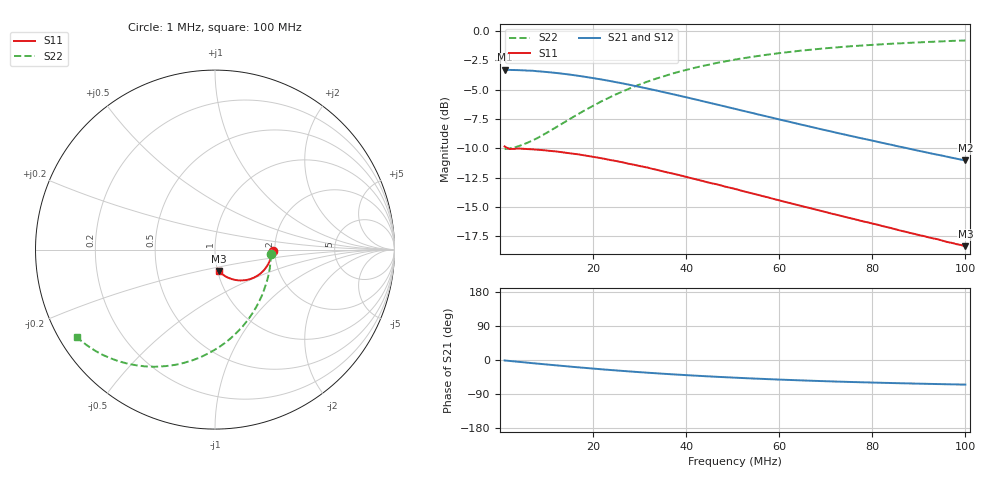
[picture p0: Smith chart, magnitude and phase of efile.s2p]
# Hz S RI R 50.0
! written by SimSmith version 18.3b
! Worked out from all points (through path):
!   101 points, 1 MHz to 100 MHz, reference 50 ohm
!   highest |S21| = -3.30 dB at 1 MHz (marker M1); lowest = -11.0 dB at 100 MHz (marker M2)
!   group delay of S21, straight-line fit = 1.73 ns
!   lowest |S11| = -18.3 dB at 100 MHz (marker M3), VSWR 1.28, Z = 50.6 - j12.3 ohm
!   |S11| at or under -10 dB: 1.736 MHz to end of sweep
!   |S22| runs from -10.1 to -0.8 dB; largest |S21 - S12| = 0.0025
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1000000  0.3221 -0.00633  0.6837 -0.0143  0.6832 -0.0144  0.3129 -0.0264
1990000  0.3138 -0.0147  0.6823 -0.0284  0.6827 -0.0285  0.3109 -0.0543
4960000  0.3129 -0.0359  0.6763 -0.0699  0.6762 -0.0699  0.2997 -0.1338
8920000  0.3046 -0.0632  0.6606 -0.1224  0.6607 -0.1226  0.2695 -0.2354
1.288e7  0.2924 -0.0879  0.6375 -0.171  0.6376 -0.1711  0.225 -0.3281
1.783e7  0.273 -0.1142  0.6001 -0.2228  0.6005 -0.2231  0.154 -0.428
2.179e7  0.2548 -0.1319  0.5661 -0.2575  0.5664 -0.2577  0.0882 -0.4937
2.575e7  0.2358 -0.1456  0.5298 -0.2847  0.53 -0.285  0.0185 -0.5458
2.872e7  0.2212 -0.1539  0.5018 -0.3009  0.5023 -0.3015  -0.0351 -0.5774
3.07e7  0.2116 -0.1583  0.4834 -0.3099  0.4834 -0.3106  -0.0703 -0.5945
3.466e7  0.1922 -0.1651  0.4467 -0.3237  0.4471 -0.3247  -0.1405 -0.621
3.862e7  0.1742 -0.1695  0.4122 -0.3328  0.4124 -0.3339  -0.2068 -0.6392
4.258e7  0.1568 -0.1712  0.3792 -0.3379  0.3794 -0.3392  -0.2706 -0.6487
4.654e7  0.141 -0.172  0.3483 -0.3397  0.3483 -0.341  -0.3294 -0.6525
5.05e7  0.1258 -0.1711  0.32 -0.3389  0.3198 -0.3402  -0.3841 -0.6507
5.446e7  0.1119 -0.1689  0.2937 -0.3361  0.2934 -0.3377  -0.4347 -0.6451
5.941e7  0.0964 -0.1651  0.2639 -0.3304  0.2634 -0.3319  -0.4916 -0.6339
6.733e7  0.075 -0.1575  0.2232 -0.3178  0.2227 -0.3195  -0.5697 -0.6099
7.525e7  0.0575 -0.1487  0.1898 -0.3032  0.1891 -0.3051  -0.6345 -0.5819
8.416e7  0.0417 -0.1383  0.1599 -0.2856  0.1585 -0.2874  -0.6925 -0.5477
9.208e7  0.0298 -0.1286  0.1374 -0.2695  0.136 -0.2715  -0.7353 -0.5165
1e8  0.0207 -0.1193  0.1192 -0.2545  0.1174 -0.256  -0.7708 -0.4869
